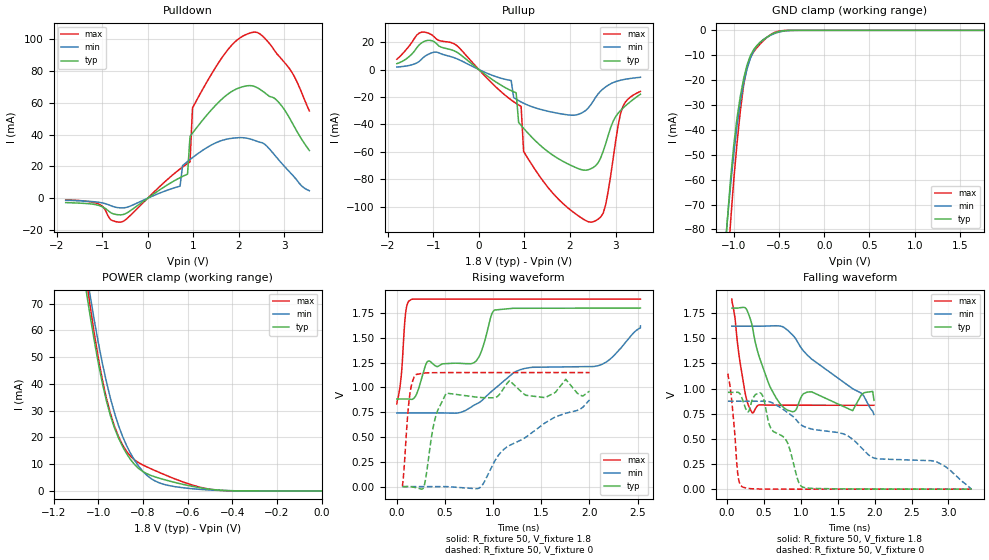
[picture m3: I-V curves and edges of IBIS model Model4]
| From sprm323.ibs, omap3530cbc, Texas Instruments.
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| Model based on original model for BQ0267CS_7LM
|   Sub model BQ0267CS_7LM_DS0_0
[model]   Model4
|[Input Load]
|[Output Drive] SLOW
|Voltage   1.8V
|Mode   I/O
Model_type   I/O
Polarity   Non-Inverting
Enable   Active-Low
Vinl =  0.6615
Vinh =  1.2285
Cref =  30.0000pF
Rref =  100.0000M
Vref =  0V
Vmeas =  0.9
C_comp   1.666797p   1.351222p   1.845128p
[Model Spec]
Vinl   0.6615   0.6615   0.6615
Vinh   1.2285   1.2285   1.2285
[Temperature Range]   25   125   -40
[Voltage Range]   1.8   1.62   1.89
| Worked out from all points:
|   slope of the pulldown table from 0 to 0.27 V, typ, clamps not added: 50.1 ohm
|   slope of the pullup table from 0 to 0.27 V, typ, clamps not added: 40.2 ohm
|   GND clamp passes 1 mA (typ) near -0.54 V on its own axis
|   POWER clamp passes 1 mA (typ) near -0.53 V on its own axis
|   rising waveform, R_fixture 50, V_fixture 1.8: 20-80 % time 701ps typ, 1.43ns min, 46.5ps max; typ from 0.883 V to 1.8 V
|   rising waveform, R_fixture 50, V_fixture 0: 20-80 % time 109ps typ, 666ps min, 55.2ps max; typ from 0 V to 0.963 V
|   falling waveform, R_fixture 50, V_fixture 1.8: 20-80 % time 213ps typ, 888ps min, 114ps max; typ from 1.8 V to 0.883 V
|   falling waveform, R_fixture 50, V_fixture 0: 20-80 % time 388ps typ, 2.12ns min, 76.8ps max; typ from 0.963 V to 0 V
[POWER_clamp]
-1.8V     610.3mA    627.2mA    665.6mA
-1.055V   75.26mA    82.88mA    80.2mA
-1.036V   65.55mA    73.22mA    69.35mA
-981.8mV  40.41mA    47.92mA    41.72mA
-963.6mV  33.78mA    40.92mA    34.77mA
-927.3mV  23.58mA    29.2mA     24.2mA
-872.7mV  13.91mA    16.92mA    14.75mA
-836.4mV  9.787mA    11.36mA    11.53mA
-781.8mV  6.423mA    5.812mA    8.958mA
-690.9mV  3.917mA    2.14mA     5.654mA
-490.9mV  560.2uA    303.2uA    525.6uA
0V        1.021nA    6.85nA     484.6pA
[Pulldown]
-1.8V     -2.78mA    -1.318mA   -1.011mA
-490.9mV  -9.78mA    -5.926mA   -13.68mA
709.1mV   12.91mA    7.574mA    18.43mA
763.6mV   13.7mA     20.47mA    19.62mA
872.7mV   15.15mA    23.06mA    21.83mA
927.3mV   38.86mA    24.31mA    22.83mA
981.8mV   40.94mA    25.53mA    56.76mA
1.691V    63.95mA    36.85mA    90.93mA
2.182V    70.72mA    37.7mA     103.3mA
2.673V    64mA       30.87mA    97.18mA
3.164V    47.7mA     14.93mA    79.19mA
3.545V    30.01mA    4.712mA    54.87mA
[Pullup]
-1.8V     4.299mA    1.801mA    7.515mA
-1.255V   19.51mA    7.643mA    27.27mA
-490.9mV  12.81mA    7.987mA    17.71mA
709.1mV   -15.4mA    -8.007mA   -22.19mA
818.2mV   -16.98mA   -21.6mA    -24.72mA
872.7mV   -38.66mA   -22.67mA   -25.85mA
927.3mV   -40.79mA   -23.66mA   -26.89mA
981.8mV   -42.88mA   -24.58mA   -59.72mA
2.455V    -72.41mA   -25.77mA   -111.4mA
2.782V    -54.15mA   -12.65mA   -98.68mA
3.164V    -28.07mA   -7.41mA    -26.66mA
3.545V    -18mA      -5.643mA   -15.97mA
[GND_clamp]
-1.8V     -558.6mA   -442.4mA   -831mA
-1.109V   -96.01mA   -92.23mA   -125.3mA
-1.073V   -76.84mA   -76.85mA   -98.77mA
-1.036V   -59.94mA   -62.48mA   -77.23mA
-1V       -45.92mA   -49.41mA   -59.83mA
-927.3mV  -26.26mA   -28.64mA   -32.16mA
-890.9mV  -19.33mA   -21.23mA   -21.91mA
-854.5mV  -14.01mA   -15.6mA    -15.01mA
-818.2mV  -10.26mA   -11.4mA    -11.04mA
-745.5mV  -6.158mA   -6.269mA   -7.023mA
-563.6mV  -1.279mA   -1.488mA   -1.068mA
1.764V    914.5pA    178nA      451pA
[Ramp]
dV/dt_f 0.62267483/0.26488767n 0.55804971/0.91064802n 0.68511618/0.12588855n
dV/dt_r 0.67239606/0.16091045n  0.5716875/0.7881303n 0.70609335/55.937014p
R_load = 50
[Rising Waveform]
R_fixture = 50
V_fixture = 1.8
V_fixture_min = 1.62
V_fixture_max = 1.89
0s        883.3mV    742.6mV    834.2mV
45.72ps   883.3mV    742.6mV    1.115V
95.29ps   883.6mV    742.6mV    1.776V
153.4ps   879mV      742.6mV    1.888V
319.8ps   1.262V     742.6mV    1.89V
824.9ps   1.268V     832.9mV    1.89V
1.014ns   1.78V      984.9mV    1.89V
1.328ns   1.798V     1.191V     1.89V
2.133ns   1.799V     1.234V     1.89V
2.529ns   1.8V       1.62V      1.89V
[Rising Waveform]
R_fixture = 50
V_fixture = 0
V_fixture_min = 0
V_fixture_max = 0
59.76ps   412.6nV    320.8nV    639.1nV
129.6ps   1.117mV    -410.2nV   886.9mV
200ps     -9.977mV   312.7nV    1.13V
282.7ps   4.441mV    -2.522uV   1.144V
390.1ps   656.7mV    -32.05uV   1.149V
513.3ps   942.6mV    527.7uV    1.149V
861.2ps   899.1mV    -10.31mV   1.15V
1.117ns   1.002V     380.6mV    1.15V
1.754ns   1.082V     740.2mV    1.15V
2ns       962.6mV    874.1mV    1.15V
[Falling Waveform]
R_fixture = 50
V_fixture = 1.8
V_fixture_min = 1.62
V_fixture_max = 1.89
64.93ps   1.8V       1.62V      1.89V
241.2ps   1.805V     1.62V      970.6mV
343.9ps   1.61V      1.62V      758.1mV
554.2ps   1.068V     1.622V     836.1mV
785.5ps   800.7mV    1.601V     834.7mV
920.9ps   779.2mV    1.504V     834.5mV
1.085ns   965.3mV    1.335V     834.4mV
1.701ns   780.2mV    998.8mV    834.2mV
1.856ns   957mV      921.3mV    834.2mV
1.99ns    883.3mV    742.6mV    834.2mV
[Falling Waveform]
R_fixture = 50
V_fixture = 0
V_fixture_min = 0
V_fixture_max = 0
11.24ps   962.6mV    874.1mV    1.15V
146.7ps   962.7mV    874.2mV    142.1mV
215ps     878mV      874.2mV    20mV
283.6ps   767mV      874.1mV    7.87mV
468.9ps   944.9mV    874.4mV    1.203mV
589.2ps   611.9mV    865.5mV    380.2uV
820.6ps   459.6mV    760.4mV    32.75uV
1.026ns   20mV       628.5mV    -1.669uV
2.844ns   494.9uV    269.9mV    -1.861uV
3.313ns   412.6nV    320.8nV    639.1nV
